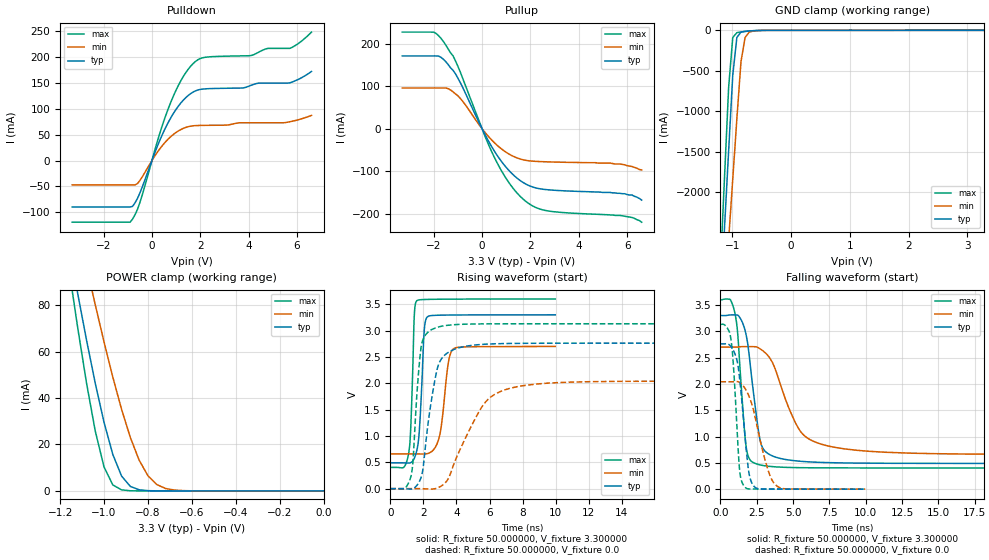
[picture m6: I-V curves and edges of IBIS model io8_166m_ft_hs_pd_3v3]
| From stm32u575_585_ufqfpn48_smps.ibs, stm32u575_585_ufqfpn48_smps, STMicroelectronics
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|   Model io8_166m_ft_hs_pd_3v3
[Model]  io8_166m_ft_hs_pd_3v3
Model_type I/O
Polarity   Non-Inverting
Enable   Active-Low
Vinl =   0.990000V
Vinh =   2.310000V
Vmeas =  1.650000V
Cref =   50.000000pF
Rref =   100.000000M
Vref =   0.0V
C_comp   3.517200pF   3.489400pF   3.557800pF
[Temperature Range]   25.000000   0.140000k   -40.000000
[Pullup Reference]   3.300000V   2.700000V   3.600000V
[Pulldown Reference]   0.0V   0.0V   0.0V
[POWER Clamp Reference]   3.300000V   2.700000V   3.600000V
[GND Clamp Reference]   0.0V   0.0V   0.0V
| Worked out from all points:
|   slope of the pulldown table from 0 to 0.495 V, typ, clamps not added: 8.73 ohm
|   slope of the pullup table from 0 to 0.495 V, typ, clamps not added: 9.64 ohm
|   GND clamp passes 1 mA (typ) near -0.50 V on its own axis
|   POWER clamp passes 1 mA (typ) near -0.85 V on its own axis
|   rising waveform, R_fixture 50.000000, V_fixture 3.300000: 20-80 % time 260ps typ, 443ps min, 195ps max; typ from 0.49 V to 3.3 V
|   rising waveform, R_fixture 50.000000, V_fixture 0.0: 20-80 % time 750ps typ, 1.95ns min, 402ps max; typ from 0 V to 2.76 V
|   falling waveform, R_fixture 50.000000, V_fixture 3.300000: 20-80 % time 759ps typ, 1.84ns min, 492ps max; typ from 3.3 V to 0.49 V
|   falling waveform, R_fixture 50.000000, V_fixture 0.0: 20-80 % time 576ps typ, 1.08ns min, 397ps max; typ from 2.76 V to 0 V
[Pulldown]
|Voltage   I(typ)   I(min)   I(max)
-3.3V     -89.72mA   -47.06mA   -119mA
-900mV    -89.72mA   -47.06mA   -119mA
-500mV    -62.92mA   -38.71mA   -81.44mA
300mV     36.2mA     21.01mA    48.7mA
800mV     84.07mA    46.96mA    114.9mA
1.3V      116.7mA    62.09mA    162.4mA
1.8V      134.4mA    67.39mA    191.2mA
2.3V      138.6mA    67.98mA    199.8mA
4.1V      145.1mA    72.79mA    202.7mA
4.8V      149.4mA    72.79mA    216.5mA
5.7V      149.8mA    74.8mA     216.5mA
6.6V      171.9mA    87.1mA     247.9mA
[Pullup]
|Voltage   I(typ)   I(min)   I(max)
-3.3V     171.2mA    95.78mA    227.3mA
-2V       171.2mA    95.78mA    227.1mA
-1.6V     163.4mA    95.78mA    205.2mA
-1.2V     137.4mA    86.68mA    171.5mA
-1V       119.2mA    77.42mA    146.9mA
100mV     -11.39mA   -7.258mA   -14.51mA
600mV     -60.65mA   -37.83mA   -77.68mA
1.2V      -103.6mA   -62.35mA   -134mA
1.8V      -129.9mA   -74.33mA   -170.6mA
2.7V      -143.6mA   -78mA      -193.2mA
5.9V      -153mA     -85mA      -206mA
6.6V      -168mA     -97mA      -220mA
[GND_clamp]
|Voltage   I(typ)   I(min)   I(max)
-3.3V     -9.098A    -9.372A    -9.671A
-1.2V     -3.386A    -4.091A    -2.933A
-1.13V    -2.437A    -3.34A     -1.815A
-1.06V    -1.49A     -2.588A    -705.6mA
-990mV    -555.7mA   -1.839A    -89.05mA
-920mV    -88.14mA   -1.093A    -28.79mA
-850mV    -22.37mA   -387.4mA   -19.86mA
-780mV    -12.13mA   -88.01mA   -13.89mA
-710mV    -7.72mA    -22.53mA   -8.86mA
-640mV    -4.556mA   -7.872mA   -4.884mA
-360mV    -39.7uA    -179.9uA   -19.45uA
3.28V     83.52uA    56.87uA    102.4uA
[POWER_clamp]
|Voltage   I(typ)   I(min)   I(max)
-3.28V    1.355A     1.167A     1.664A
-1.16V    105.7mA    131.6mA    95.69mA
-1.12V    84.97mA    114mA      70.27mA
-1.08V    65.05mA    96.83mA    46.54mA
-1.04V    46.34mA    80.15mA    25.76mA
-1V       29.51mA    64.13mA    10.3mA
-960mV    15.69mA    48.99mA    2.571mA
-920mV    6.373mA    35.1mA     455.6uA
-840mV    490.7uA    13.24mA    11.36uA
-760mV    27.33uA    2.767mA    278.3nA
-640mV    347.6nA    134.1uA    16.77nA
0V        0A         19.95nA    0A
[Ramp]
| variable   typ   min   max
dV/dt_r  1.65672/0.74842n   1.22418/1.94747n   1.87812/0.40096n
dV/dt_f  1.68577/0.75769n   1.22332/1.83445n   1.91752/0.48996n
R_load = 50.000000
[Rising Waveform]
R_fixture= 50.000000
V_fixture= 3.300000
V_fixture_min= 2.700000
V_fixture_max= 3.600000
|time   V(typ)   V(min)   V(max)
0s        489.8mV    659.5mV    403.4mV
1.121ns   485.5mV    659.5mV    691.4mV
1.261ns   497.5mV    659.5mV    1.342V
1.461ns   581.8mV    659.4mV    3.343V
1.602ns   720.9mV    659.3mV    3.566V
2.062ns   3.036V     657.7mV    3.59V
2.242ns   3.261V     664.6mV    3.592V
2.983ns   3.292V     1.007V     3.596V
3.844ns   3.296V     2.659V     3.597V
9.97ns    3.299V     2.699V     3.599V
[Rising Waveform]
R_fixture= 50.000000
V_fixture= 0.0
V_fixture_min= 0.0
V_fixture_max= 0.0
|time   V(typ)   V(min)   V(max)
0s        3.582uV    4.866uV    1.477uV
1.251ns   -9.839mV   38.92uV    236.3mV
1.351ns   -4.936mV   55.1uV     437.7mV
1.602ns   59.61mV    134.5uV    1.76V
1.852ns   202.2mV    -413.1uV   2.663V
2.753ns   2.152V     2.386mV    3.053V
3.504ns   2.586V     190.8mV    3.102V
5.606ns   2.739V     1.582V     3.127V
7.207ns   2.756V     1.902V     3.129V
24.92ns   2.761V     2.04V      3.13V
[Falling Waveform]
R_fixture= 50.000000
V_fixture= 3.300000
V_fixture_min= 2.700000
V_fixture_max= 3.600000
|time   V(typ)   V(min)   V(max)
0s        3.299V     2.699V     3.599V
1.001ns   3.311V     2.699V     3.341V
1.201ns   3.306V     2.702V     2.923V
1.752ns   2.958V     2.709V     842.1mV
2.302ns   1.772V     2.708V     500.9mV
2.703ns   970.3mV    2.672V     463.1mV
3.103ns   713.5mV    2.586V     442.4mV
5.355ns   534.1mV    1.163V     409.2mV
6.957ns   508.4mV    853.6mV    405.4mV
24.92ns   489.8mV    659.5mV    403.4mV
[Falling Waveform]
R_fixture= 50.000000
V_fixture= 0.0
V_fixture_min= 0.0
V_fixture_max= 0.0
|time   V(typ)   V(min)   V(max)
0s        2.761V     2.04V      3.13V
720.7ps   2.711V     2.04V      2.853V
920.9ps   2.62V      2.041V     2.243V
1.321ns   2.102V     2.03V      363.1mV
1.662ns   1.101V     1.927V     45.85mV
1.942ns   349mV      1.784V     4.914mV
2.202ns   96.54mV    1.581V     2.997mV
3.203ns   2.555mV    431.3mV    1.295mV
3.904ns   1.532mV    57.03mV    888.8uV
9.97ns    3.582uV    4.866uV    1.477uV
